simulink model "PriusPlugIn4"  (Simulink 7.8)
settings: Solver=ode23t  StartTime=0.0  StopTime=1180  MaxStep=0.01  RelTol=1e-3
InitFcn:
  | init_Prius_GT
StopFcn:
  | Vyhodnoceni
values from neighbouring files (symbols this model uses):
  k = Nr/Ns    (= 2.6)    [init_Prius_GT.m]
  Mpr = Nr/(Nr+Ns)    (= 0.722222222222)    [init_Prius_GT.m]
  Mps = Ns/(Nr+Ns)    (= 0.277777777778)    [init_Prius_GT.m]
  om_diff_ic = 0    [init_Prius_GT.m]
  omric = 0    [init_Prius_GT.m]
  rpm_FMEP = [1,500,1000,1500,2000,2500,3000,3500,4000,4500,5000]    [init_Prius_GT.m]
  t_sample = 0.1    [init_Prius_GT.m]
  torque_FMEP = [0,0,0.58,0.66,0.75,0.84,0.93,1.1,1.3,1.4,1.5].*(Vdis/(4*pi))*100000    [init_Prius_GT.m]
  vf0 = 0    [init_Prius_GT.m]
undefined symbols (not defined in the file or in its folder): Battery, Battery_Pack, Clutch, Differential, Driveshaft, Engine, Environment, Gearbox, Motor, Powertrain, table_FMEP, Vehicle
libraries: simulink x24, simulink_extras x4, simulink_need_slupdate x1
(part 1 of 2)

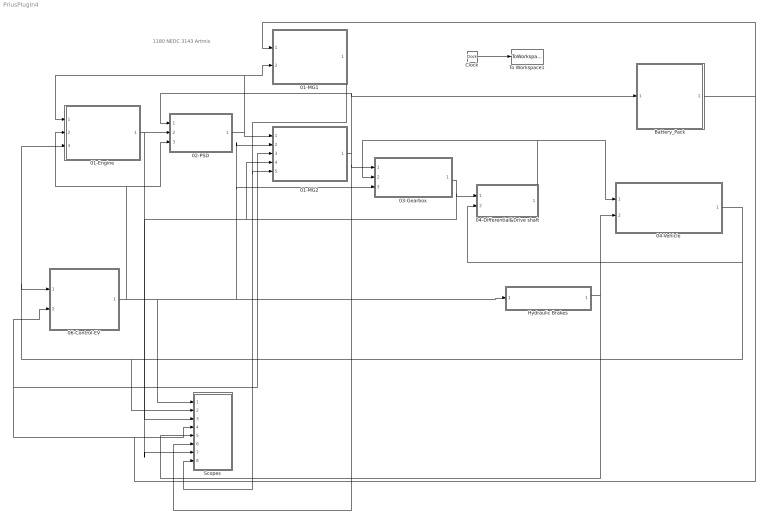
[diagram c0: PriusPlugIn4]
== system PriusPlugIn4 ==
  note: 1180 NEDC 3143 Artmis
  01-Engine : Subsystem  AncestorBlock=Powertrain/01-Engine
  01-MG1 : Subsystem  AncestorBlock=Powertrain/Electric Drive
  01-MG2 : Subsystem  AncestorBlock=Powertrain/Electric Drive
  02-PSD : Subsystem  AncestorBlock=Powertrain/02-Clutch
  03-Gearbox : Subsystem  AncestorBlock=Powertrain/03-Gearbox
  04-Differential&Drive shaft : Subsystem  AncestorBlock=Powertrain/04-Differential&Drive shaft
  04-Vehicle : Subsystem  AncestorBlock=Powertrain/05-Vehicle
  06-Control-EV : Subsystem
  Battery_Pack : Subsystem  AncestorBlock=Powertrain/Battery_Pack
  Clock : Clock
  Hydraulic Brakes : Subsystem  AncestorBlock=Powertrain/Hydraulic Brakes  TreatAsAtomicUnit=on
  Scopes : Subsystem
  To Workspace1 : ToWorkspace  VariableName=t  SampleTime=t_sample  SaveFormat=Array
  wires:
  03-Gearbox/1(BUS_Gearbox) -> 04-Differential&Drive shaft/1(BUS_Gearbox), Scopes/3(BUS_Gearbox), 01-MG2/4(BUS_Gearbox)
  04-Differential&Drive shaft/1(BUS_Driveshaft) -> 03-Gearbox/2(BUS_Driveshaft), 04-Vehicle/1(BUS_Driveshaft_Front)
  06-Control-EV/1(BUS_Control) -> Scopes/1(BUS_Control), 03-Gearbox/3(BUS_Control), 01-MG2/2(BUS_Control), Hydraulic Brakes/1(BUS_Control), 01-Engine/2(BUS_Control), 02-PSD/3(BUS_Control)
  04-Vehicle/1(BUS_Vehicle) -> 04-Differential&Drive shaft/2(BUS_Vehicle), Scopes/2(BUS_Vehicle), 06-Control-EV/1(BUS_Vehicle), 01-Engine/3(BUS_vehicle)
  Battery_Pack/1(BUS_Battery) -> Scopes/4(BUS_Battery), 06-Control-EV/2(BUS_Battery), 01-MG2/3(BUS_Battery), 01-MG1/1(BUS_Battery)
  Hydraulic Brakes/1(BUS_Brakes) -> Scopes/5(BUS_Brakes), 04-Vehicle/2(BUS_Brakes)
  01-Engine/1(BUS_Engine) -> 02-PSD/2(BUS_Engine), Scopes/7(BUS_Engine)
  02-PSD/1(BUS_PSD) -> 01-MG2/1(BUS_PSD), 01-Engine/1(BUS_PSD), 01-MG1/2(BUS_PSD)
  01-MG2/1(BUS_MG2) -> 02-PSD/1(BUS_MG2), Battery_Pack/1(BUS_MG2), 03-Gearbox/1(BUS_MG2), Scopes/6(BUS_Motor)
  01-MG1/1(BUS_MG1) -> 01-MG2/5(BUS_MG1), Scopes/8(BUS_MG1)
  Clock/1 -> To Workspace1/1

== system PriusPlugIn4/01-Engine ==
  BUS_PSD : Inport
  BUS_Control : Inport  Port=2
  BUS_vehicle : Inport  Port=3
  1-D Lookup Table : Lookup_n-D  NumberOfTableDimensions=1  BreakpointsForDimension1=[1000,1625,2250,3000,3750,4500,5250,5625]  Table=[85,90,100,112,100,92,85,78]  RndMeth=Simplest
  Bus Creator : BusCreator  Inputs=6
  Bus Selector : BusSelector  OutputSignals=om_c
  Bus Selector1 : BusSelector  OutputSignals=Throttle_Engine[-],Throttle_excd,Mode
  Bus Selector2 : BusSelector  OutputSignals=s_veh
  Consumption/Emissions : Subsystem
  Display : Display
  Mechanical : Subsystem
  Mux : Mux  Inputs=2
  Product2 : Product
  Saturation : Saturate  UpperLimit=inf  LowerLimit=0
  Scope : Scope  NumInputPorts=3
  Scope1 : Scope
  rad2rpm : Gain  Gain=30/pi
  BUS_Engine : Outport
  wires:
  Product2/1 -> Mux/1, Mechanical/1(Te_dem), Scope/3
  1-D Lookup Table/1 -> Product2/1
  Bus Selector1/1 -> Scope/1, Product2/2  "<Throttle_Engine[-]>"
  Consumption/Emissions/2(Fuel_cons_m) -> Bus Creator/5  "Fuel_cons_m"
  Saturation/1 -> Consumption/Emissions/2(Pe)
  Consumption/Emissions/1(Fuel_cons) -> Bus Creator/4  "fuel_cons [l_100km]"
  Bus Selector2/1 -> Display/1, Consumption/Emissions/3(s)  "<s_veh>"
  BUS_vehicle/1 -> Bus Selector2/1
  BUS_Control/1 -> Bus Selector1/1
  Bus Selector/1 -> Mechanical/2(om_fric)  "<om_c>"
  BUS_PSD/1 -> Bus Selector/1
  Bus Creator/1 -> BUS_Engine/1
  Mechanical/3(Tec) -> Mux/2, Consumption/Emissions/4(Te), Bus Creator/3  "Teng [Nm]"
  Mechanical/2(Pe) -> Saturation/1, Bus Creator/2  "Pe[kW]"
  Mechanical/1(om_e) -> rad2rpm/1
  rad2rpm/1 -> 1-D Lookup Table/1, Scope/2, Bus Creator/1, Consumption/Emissions/1(n_eng[rpm])  "n_eng[rpm]"
  Mechanical/4(Pe_dem) -> Bus Creator/6  "Pe_dem[kW]"
  Bus Selector1/2 -> Mechanical/3(Multip)  "<Throttle_excd>"
  Mux/1 -> Scope1/1

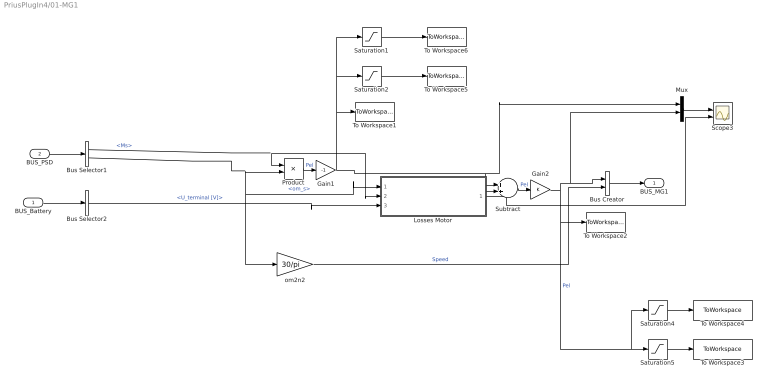
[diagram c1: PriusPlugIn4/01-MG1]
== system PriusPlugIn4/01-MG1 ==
  BUS_Battery : Inport
  BUS_PSD : Inport  Port=2
  Bus Creator : BusCreator  Inputs=2
  Bus Selector1 : BusSelector  OutputSignals=Ms,om_s
  Bus Selector2 : BusSelector  OutputSignals=U_terminal [V]
  Gain1 : Gain  Gain=-1
  Gain2 : Gain
  Losses Motor : Subsystem
  Mux : Mux  Inputs=2
  Product : Product
  Saturation1 : Saturate  UpperLimit=0  LowerLimit=-inf
  Saturation2 : Saturate  UpperLimit=inf  LowerLimit=0
  Saturation4 : Saturate  UpperLimit=0  LowerLimit=-inf
  Saturation5 : Saturate  UpperLimit=inf  LowerLimit=0
  Scope3 : Scope  NumInputPorts=2
  Subtract : Sum
  To Workspace1 : ToWorkspace  VariableName=P_MG1  SampleTime=t_sample  SaveFormat=Array
  To Workspace2 : ToWorkspace  VariableName=P_MG1el  SampleTime=t_sample  SaveFormat=Array
  To Workspace3 : ToWorkspace  VariableName=P_MG1el_mot  SampleTime=t_sample  SaveFormat=Array
  To Workspace4 : ToWorkspace  VariableName=P_MG1el_gen  SampleTime=t_sample  SaveFormat=Array
  To Workspace5 : ToWorkspace  VariableName=P_MG1mech_mot  SampleTime=t_sample  SaveFormat=Array
  To Workspace6 : ToWorkspace  VariableName=P_MG1mech_gen  SampleTime=t_sample  SaveFormat=Array
  om2n2 : Gain  Gain=30/pi
  BUS_MG1 : Outport
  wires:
  BUS_Battery/1 -> Bus Selector2/1
  BUS_PSD/1 -> Bus Selector1/1
  Bus Selector1/1 -> Losses Motor/2(Torque), Product/1  "<Ms>"
  Bus Selector1/2 -> Losses Motor/1(Speed), om2n2/1, Product/2  "<om_s>"
  Product/1 -> Gain1/1  "Pel"
  Bus Creator/1 -> BUS_MG1/1
  Subtract/1 -> Gain2/1  "Pel"
  Losses Motor/1(P_loss) -> Scope3/2, Subtract/2
  Gain1/1 -> Saturation1/1, Saturation2/1, To Workspace1/1, Mux/1, Subtract/1
  om2n2/1 -> Bus Creator/2  "Speed"
  Saturation4/1 -> To Workspace4/1
  Saturation5/1 -> To Workspace3/1
  Saturation1/1 -> To Workspace6/1
  Saturation2/1 -> To Workspace5/1
  Mux/1 -> Scope3/1
  Bus Selector2/1 -> Losses Motor/3(Voltage [V])  "<U_terminal [V]>"
  Gain2/1 -> Mux/2, Bus Creator/1, Saturation4/1, Saturation5/1, To Workspace2/1  "Pel"

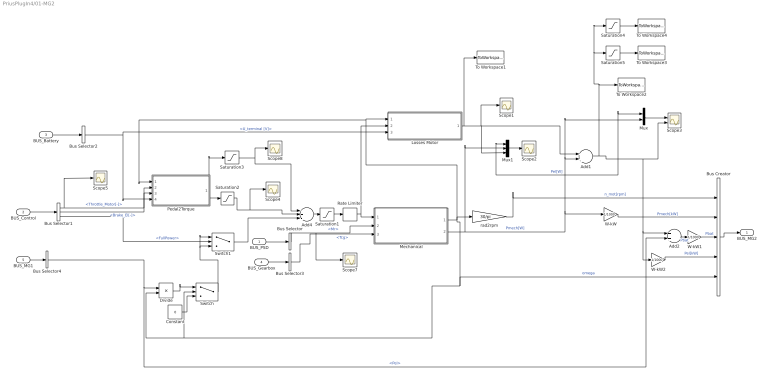
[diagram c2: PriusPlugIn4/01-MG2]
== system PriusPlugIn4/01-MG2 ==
  BUS_PSD : Inport
  BUS_Control : Inport  Port=2
  BUS_Battery : Inport  Port=3
  BUS_Gearbox : Inport  Port=4
  BUS_MG1 : Inport  Port=5
  Add1 : Sum
  Add2 : Sum
  Add4 : Sum  Inputs=++-
  Bus Creator : BusCreator  Inputs=5
  Bus Selector : BusSelector  OutputSignals=Mr
  Bus Selector1 : BusSelector  OutputSignals=Throttle_Motor[-],Brake_El[-],FullPower
  Bus Selector2 : BusSelector  OutputSignals=U_terminal [V]
  Bus Selector3 : BusSelector  OutputSignals=Tcg
  Bus Selector4 : BusSelector  OutputSignals=Pel
  Constant : Constant  Value=0
  Divide : Product  Inputs=*/
  Losses Motor : Subsystem
  Mechanical : Subsystem
  Mux : Mux  Inputs=2
  Mux1 : Mux  Inputs=3
  Pedal2Torque : Subsystem
  Rate Limiter : RateLimiter  RisingSlewLimit=100  FallingSlewLimit=-100  SampleTimeMode=inherited
  Saturation1 : Saturate  UpperLimit=500  LowerLimit=-500
  Saturation2 : Saturate  UpperLimit=inf  LowerLimit=0
  Saturation3 : Saturate  UpperLimit=0  LowerLimit=-inf
  Saturation4 : Saturate  UpperLimit=0  LowerLimit=-inf
  Saturation5 : Saturate  UpperLimit=inf  LowerLimit=0
  Scope{1..2,4..5,7..8} (6 alike) : Scope
  Scope3 : Scope  NumInputPorts=2
  Switch : Switch  Threshold=3
  Switch1 : Switch  Threshold=1
  To Workspace1 : ToWorkspace  VariableName=P_MG2_loss  SampleTime=t_sample  SaveFormat=Array
  To Workspace2 : ToWorkspace  VariableName=P_MG2el  SampleTime=t_sample  SaveFormat=Array
  To Workspace3 : ToWorkspace  VariableName=P_MG2el_mot  SampleTime=t_sample  SaveFormat=Array
  To Workspace4 : ToWorkspace  VariableName=P_MG2el_gen  SampleTime=t_sample  SaveFormat=Array
  W-kW : Gain  Gain=1/1000
  W-kW1 : Gain  Gain=1/1000
  W-kW2 : Gain  Gain=1/1000
  rad2rpm : Gain  Gain=30/pi
  BUS_MG2 : Outport
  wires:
  W-kW2/1 -> Bus Creator/4  "Pel[kW]"
  W-kW/1 -> Bus Creator/2  "Pmech[kW]"
  Bus Selector1/2 -> Pedal2Torque/3(Brake_el[-])  "<Brake_El[-]>"
  Bus Selector1/1 -> Pedal2Torque/2(Throttle_pedal[-]), Scope5/1  "<Throttle_Motor[-]>"
  BUS_Control/1 -> Bus Selector1/1
  BUS_PSD/1 -> Bus Selector/1
  Bus Creator/1 -> BUS_MG2/1
  Mechanical/2(Pmech) -> W-kW/1, Mux/2, Add1/2, Mux1/2  "Pmech[W]"
  Mechanical/1(om_e) -> Divide/2, Switch/2, Bus Creator/5, rad2rpm/1, Losses Motor/1(Speed), Pedal2Torque/1(om_motor)  "omega"
  rad2rpm/1 -> Bus Creator/1  "n_mot[rpm]"
  BUS_Battery/1 -> Bus Selector2/1
  Bus Selector2/1 -> Losses Motor/3(Voltage [V]), Pedal2Torque/4(Voltage [V])  "<U_terminal [V]>"
  Losses Motor/1(P_loss) -> To Workspace1/1, Mux1/3, Add1/1, Scope1/1
  BUS_Gearbox/1 -> Bus Selector3/1
  Bus Selector3/1 -> Mechanical/3(Tcg)  "<Tcg>"
  Bus Selector/1 -> Mechanical/2(Tr), Scope7/1  "<Mr>"
  BUS_MG1/1 -> Bus Selector4/1
  Add1/1 -> To Workspace2/1, Saturation4/1, Saturation5/1, Mux1/1, Mux/1, Scope3/2, Add2/1, W-kW2/1  "Pel[W]"
  Mux/1 -> Scope3/1
  Pedal2Torque/1(Te) -> Saturation2/1, Saturation3/1
  Saturation3/1 -> Add4/1, Scope8/1
  Add4/1 -> Saturation1/1
  Saturation2/1 -> Add4/2, Scope4/1
  Saturation1/1 -> Rate Limiter/1
  Bus Selector4/1 -> Add2/2, Divide/1  "<Pel>"
  Constant/1 -> Switch/3
  Divide/1 -> Switch/1
  Bus Selector1/3 -> Switch1/2  "<FullPower>"
  Switch/1 -> Switch1/3, Switch1/1
  Switch1/1 -> Add4/3
  Rate Limiter/1 -> Mechanical/1(T_MG2), Losses Motor/2(Torque)
  Add2/1 -> W-kW1/1  "Pbat"
  W-kW1/1 -> Bus Creator/3  "Pbat"
  Mux1/1 -> Scope2/1
  Saturation4/1 -> To Workspace4/1
  Saturation5/1 -> To Workspace3/1

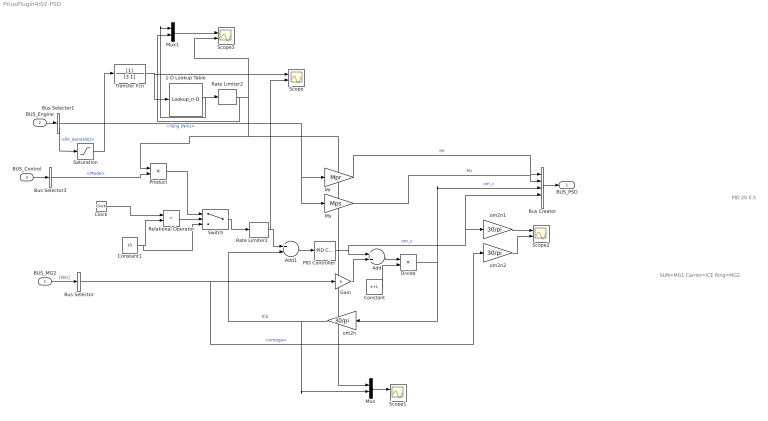
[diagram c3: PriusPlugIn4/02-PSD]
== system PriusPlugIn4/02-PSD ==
  note: SUN=MG1 Carrier=ICE Ring=MG2
  note: PID 20 0.5
  BUS_MG2 : Inport
  BUS_Engine : Inport  Port=2
  BUS_Control : Inport  Port=3
  1-D Lookup Table : Lookup_n-D  NumberOfTableDimensions=1  BreakpointsForDimension1=|  Table=|  RndMeth=Simplest
      | [0
      | 1000
      | 7891
      | 19181
      | 30174
      | 42286
      | 54998]/1000
      | [0
      | 1150
      | 1155
      | 2000
      | 2750
      | 3500
      | 4250]
  Add : Sum
  Add1 : Sum  Inputs=+-
  Bus Creator : BusCreator  Inputs=5
  Bus Selector : BusSelector  OutputSignals=omega
  Bus Selector1 : BusSelector  OutputSignals=n_eng[rpm],Teng [Nm],Pe_dem[kW]
  Bus Selector3 : BusSelector  OutputSignals=Mode
  Clock : Clock
  Constant : Constant  Value=k+1
  Constant1 : Constant  Value=10
  Divide : Product  Inputs=*/
  Gain : Gain  Gain=k
  Mr : Gain  Gain=Mpr
  Ms : Gain  Gain=Mps
  Mux : Mux  Inputs=2
  Mux1 : Mux  Inputs=2
  PID Controller : simulink/Continuous/PID Controller  Controller=PID  TimeDomain=Continuous-time  SampleTime=1  IntegratorMethod=Forward Euler  FilterMethod=Forward Euler  Form=Parallel  P=20  I=0.5*10  D=0  N=0  InitialConditionSource=internal  InitialConditionForIntegrator=0  InitialConditionForFilter=0  ExternalReset=none  LimitOutput=off  UpperSaturationLimit=6500/30*pi  LowerSaturationLimit=-6500/30*pi  LinearizeAsGain=off  AntiWindupMode=none  Kb=1  TrackingMode=off  Kt=1  PParamMin=[]  PParamMax=[]  IParamMin=[]  IParamMax=[]  DParamMin=[]  DParamMax=[]  NParamMin=[]  NParamMax=[]  KbParamMin=[]  KbParamMax=[]  KtParamMin=[]  KtParamMax=[]  POutMin=[]  POutMax=[]  IOutMin=[]  IOutMax=[]  DOutMin=[]  DOutMax=[]  NOutMin=[]  NOutMax=[]  KbOutMin=[]  KbOutMax=[]  KtOutMin=[]  KtOutMax=[]  IntegratorOutMin=[]  IntegratorOutMax=[]  FilterOutMin=[]  FilterOutMax=[]  SumOutMin=[]  SumOutMax=[]  SumI1OutMin=[]  SumI1OutMax=[]  SumI2OutMin=[]  SumI2OutMax=[]  SumI3OutMin=[]  SumI3OutMax=[]  SumDOutMin=[]  SumDOutMax=[]  SaturationOutMin=[]  SaturationOutMax=[]  IntegratorContinuousStateAttributes=''  IntegratorStateMustResolveToSignalObject=off  IntegratorRTWStateStorageClass=Auto  FilterContinuousStateAttributes=''  FilterStateMustResolveToSignalObject=off  FilterRTWStateStorageClass=Auto
  Product : Product
  Rate Limiter1 : RateLimiter  RisingSlewLimit=300  FallingSlewLimit=-300
  Rate Limiter2 : RateLimiter  RisingSlewLimit=500  FallingSlewLimit=-500
  Relational Operator : RelationalOperator  Operator=>  OutDataTypeStr=boolean
  Saturation : Saturate  UpperLimit=47  LowerLimit=0
  Scope{,1..3} (4 alike) : Scope  NumInputPorts=2
  Switch : Switch
  Transfer Fcn : TransferFcn  Denominator=[3 1]
  om2n : Gain  Gain=30/pi
  om2n1 : Gain  Gain=30/pi
  om2n2 : Gain  Gain=30/pi
  BUS_PSD : Outport
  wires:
  BUS_Engine/1 -> Bus Selector1/1
  Bus Creator/1 -> BUS_PSD/1
  BUS_MG2/1 -> Bus Selector/1  "[Nm]"
  BUS_Control/1 -> Bus Selector3/1
  Bus Selector1/2 -> Mr/1, Ms/1  "<Teng [Nm]>"
  PID Controller/1 -> Add/1, Bus Creator/4, om2n1/1  "om_s"
  Gain/1 -> Add/2
  Add/1 -> Divide/1
  Constant/1 -> Divide/2
  Divide/1 -> Bus Creator/3, om2n/1  "om_c"
  Mr/1 -> Bus Creator/1  "Mr"
  om2n/1 -> Add1/2, Mux/2  "ICE"
  Add1/1 -> PID Controller/1
  Ms/1 -> Bus Creator/2  "Ms"
  Bus Selector/1 -> Gain/1, om2n2/1  "<omega>"
  Constant1/1 -> Relational Operator/2, Switch/3
  Clock/1 -> Relational Operator/1
  Relational Operator/1 -> Switch/2
  Switch/1 -> Rate Limiter1/1
  Bus Selector1/3 -> Saturation/1  "<Pe_dem[kW]>"
  1-D Lookup Table/1 -> Mux1/1, Rate Limiter2/1
  Mux/1 -> Scope1/1
  Product/1 -> Switch/1
  Rate Limiter1/1 -> Add1/1, Scope/2
  om2n1/1 -> Scope2/1
  om2n2/1 -> Scope2/2
  Bus Selector3/1 -> Product/2  "<Mode>"
  Saturation/1 -> Transfer Fcn/1
  Mux1/1 -> Scope3/1
  Rate Limiter2/1 -> Mux1/2, Product/1, Mux/1, Scope3/2
  Transfer Fcn/1 -> Scope/1, 1-D Lookup Table/1

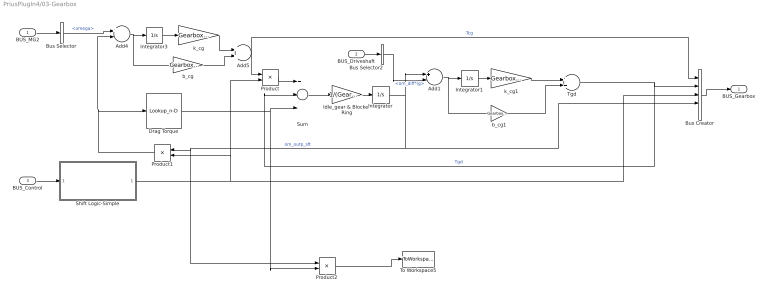
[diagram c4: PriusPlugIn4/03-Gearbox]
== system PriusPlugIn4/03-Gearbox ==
  BUS_MG2 : Inport
  BUS_Driveshaft : Inport  Port=2
  BUS_Control : Inport  Port=3
  Add1 : Sum  Inputs=+-
  Add4 : Sum  Inputs=+-
  Add5 : Sum
  Bus Creator : BusCreator  Inputs=5
  Bus Selector : BusSelector  OutputSignals=omega
  Bus Selector2 : BusSelector  OutputSignals=om_diff*ig
  Drag Torque : Lookup_n-D  NumberOfTableDimensions=1  BreakpointsForDimension1=[0 100 200 300 400]  Table=[0 1 2 3 3.5]  RndMeth=Simplest
  Idle_gear & Blocker Ring : Gain  Gain=1/(Gearbox.Inpsft.Inertia+Gearbox.Outpsft.Inertia)
  Integrator : Integrator
  Integrator1 : Integrator
  Integrator3 : Integrator
  Product : Product
  Product1 : Product
  Product2 : Product
  Shift Logic-Simple : Subsystem
  Sum : Sum  Inputs=+--
  Tgd : Sum
  To Workspace5 : ToWorkspace  VariableName=P_Gearbox  SampleTime=t_sample  SaveFormat=Array
  b_cg : Gain  Gain=Gearbox.Inpsft.b
  b_cg1 : Gain  Gain=Gearbox.Outpsft.b
  k_cg : Gain  Gain=Gearbox.Inpsft.c
  k_cg1 : Gain  Gain=Gearbox.Outpsft.c
  BUS_Gearbox : Outport
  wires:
  Bus Selector2/1 -> Add1/2  "<om_diff*ig>"
  BUS_Driveshaft/1 -> Bus Selector2/1
  Tgd/1 -> Bus Creator/2, Sum/2  "Tgd"
  Add1/1 -> b_cg1/1, Integrator1/1
  Integrator1/1 -> k_cg1/1
  k_cg1/1 -> Tgd/1
  b_cg1/1 -> Tgd/2
  Shift Logic-Simple/1(Gear_ratio) -> Bus Creator/3, Product1/2, Product/2
  Bus Creator/1 -> BUS_Gearbox/1
  BUS_Control/1 -> Shift Logic-Simple/1(BUS_Control)
  Bus Selector/1 -> Add4/1  "<omega>"
  BUS_MG2/1 -> Bus Selector/1
  Product1/1 -> Drag Torque/1, Add4/2
  Product/1 -> Sum/1
  b_cg/1 -> Add5/2
  k_cg/1 -> Add5/1
  Integrator3/1 -> k_cg/1
  Add4/1 -> Integrator3/1, b_cg/1
  Integrator/1 -> Add1/1, Product2/1, Product1/1, Bus Creator/4  "om_outp_sft"
  Idle_gear & Blocker Ring/1 -> Integrator/1
  Sum/1 -> Idle_gear & Blocker Ring/1
  Add5/1 -> Bus Creator/1, Product/1  "Tcg"
  Product2/1 -> To Workspace5/1
  Drag Torque/1 -> Product2/2, Sum/3

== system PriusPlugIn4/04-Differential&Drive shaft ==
  BUS_Gearbox : Inport
  BUS_Vehicle : Inport  Port=2
  Bus Creator : BusCreator  Inputs=2
  Bus Selector2 : BusSelector  OutputSignals=Tgd
  Differential : Subsystem
  Driveshafts : Subsystem
  BUS_Driveshaft : Outport
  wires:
  Driveshafts/1(T_drvsft) -> Differential/2(T_drv_sft), Bus Creator/1
  Differential/2(om_diff*ig) -> Bus Creator/2  "om_diff*ig"
  Bus Selector2/1 -> Differential/1(Tgd)  "<Tgd>"
  Differential/1(om_diff) -> Driveshafts/1(om_diff)
  BUS_Vehicle/1 -> Driveshafts/2(BUS_Vehicle)
  Bus Creator/1 -> BUS_Driveshaft/1
  BUS_Gearbox/1 -> Bus Selector2/1

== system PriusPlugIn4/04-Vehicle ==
  BUS_Driveshaft_Front : Inport
  BUS_Brakes : Inport  Port=2
  "          1" : Product  Inputs=**
  "          2" : Product  Inputs=**
  Add : Sum
  Bus Creator : BusCreator  Inputs=5
  Bus Selector1 : BusSelector  OutputSignals=T_drvsft
  Bus Selector3 : BusSelector  OutputSignals=Brakes_Front,Brakes_Rear
  Dynamics : Subsystem
  Subtract2 : Sum
  Tire front : Subsystem
  Tire rear : Subsystem
  To Workspace2 : ToWorkspace  VariableName=P_brakes  SampleTime=t_sample  SaveFormat=Array
  Weight distribution : Subsystem
  BUS_Vehicle : Outport
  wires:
  "          2"/1 -> Subtract2/2
  Subtract2/1 -> To Workspace2/1
  "          1"/1 -> Subtract2/1
  Bus Selector3/2 -> Tire rear/2(T_drsft), "          2"/2  "<Brakes_Rear>"
  Bus Selector3/1 -> "          1"/2, Add/2  "<Brakes_Front>"
  BUS_Brakes/1 -> Bus Selector3/1
  Bus Selector1/1 -> Add/1  "<T_drvsft>"
  Add/1 -> Tire front/2(T_drsft)
  Dynamics/2(s_veh) -> Bus Creator/2  "s_veh"
  Tire front/1(F_tire) -> Dynamics/1(F_tire_front)
  Tire rear/1(F_tire) -> Dynamics/2(F_tire_rear)
  BUS_Driveshaft_Front/1 -> Bus Selector1/1
  Bus Creator/1 -> BUS_Vehicle/1
  Weight distribution/1(Fn_Wheel_F) -> Dynamics/3(Fn_Wheel_F)
  Weight distribution/2(Fn_Wheel_R) -> Dynamics/4(Fn_Wheel_R)
  Dynamics/1(v_veh) -> Bus Creator/1  "v_veh"
  Dynamics/3(v_f[m/s]) -> Tire front/1(v_f), Tire rear/1(v_f)
  Dynamics/4(Acc) -> Bus Creator/5, Weight distribution/1(acc)  "a_veh"
  Tire front/2(om_wheel) -> "          1"/1, Bus Creator/3  "om_wheel_f"
  Tire rear/2(om_wheel) -> "          2"/1, Bus Creator/4  "om_wheel_r"

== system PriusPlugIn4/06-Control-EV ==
  BUS_Vehicle : Inport
  BUS_Battery : Inport  Port=2
  Brakes : Scope  NumInputPorts=5
  Bus Creator : BusCreator  Inputs=10
  Bus Selector1 : BusSelector  OutputSignals=SOC[%]
  Bus Selector2 : BusSelector  OutputSignals=v_veh,a_veh
  Cockpit : Subsystem
  Constant : Constant  Value=0
  Cycle : Subsystem
  Driver : Subsystem
  Electric : Subsystem
  Full Power : Subsystem
  Gain : Gain  Gain=0
  Hybrid : Subsystem
  Manual Switch : simulink/Signal Routing/Manual Switch  sw=0  action=0  varsize=off
  BUS_Control : Outport
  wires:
  Cockpit/2(Clutch1) -> Bus Creator/2  "Clutch_pedal[-]"
  Cockpit/1(ThrottleEngine) -> Bus Creator/1  "Throttle_Engine[-]"
  Cockpit/3(BrakeEl) -> Bus Creator/3  "Brake_El[-]"
  Driver/1(Throttle [Nm]) -> Cockpit/1(Throttle_in), Electric/3(Throttle), Hybrid/3(Throttle), Full Power/3(Throttle)
  Driver/2(Brake [Nm]) -> Cockpit/2(Brake)
  Cycle/2(v_dem [-]) -> Bus Creator/5, Driver/2(v_dem [km/h])  "v_dem[kmh]"
  Cycle/1(Gear_dem [-]) -> Bus Creator/4  "Gear[-]"
  Bus Creator/1 -> BUS_Control/1
  BUS_Vehicle/1 -> Bus Selector2/1
  Bus Selector2/1 -> Cockpit/4(v-veh), Driver/1(v_veh [km/h]), Hybrid/1(In1), Full Power/1(In1), Electric/1(v_veh)  "<v_veh>"
  Bus Selector2/2 -> Cockpit/3(a-veh)  "<a_veh>"
  Cockpit/4(BrakeHyd) -> Bus Creator/6  "Brake_Hyd[-]"
  Cockpit/5(ThrottleMotor) -> Bus Creator/7  "Throttle_Motor[-]"
  BUS_Battery/1 -> Bus Selector1/1
  Bus Selector1/1 -> Electric/2(SOC), Hybrid/2(SOC), Full Power/2(SOC)  "<SOC[%]>"
  Electric/1(Out1) -> Brakes/1  "Electric"
  Hybrid/1(Out1) -> Brakes/2, Manual Switch/2  "Mode"
  Full Power/1(Out1) -> Gain/1  "FullPower"
  Driver/3(Throttle_excd) -> Bus Creator/10  "Throttle_excd"
  Manual Switch/1 -> Cockpit/5(Mode), Bus Creator/8  "Mode"
  Constant/1 -> Manual Switch/1
  Gain/1 -> Cockpit/6(FullPower), Brakes/3, Bus Creator/9  "FullPower"

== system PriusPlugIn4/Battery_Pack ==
  BUS_MG2 : Inport
  Bus Creator : BusCreator  Inputs=5
  Bus Selector : BusSelector  OutputSignals=Pbat
  Cell : Subsystem
  Divide : Product  Inputs=*/
  Divide1 : Product  Inputs=*/
  Gain1 : Gain  Gain=1000
  Memory1 : Memory  X0=400
  Memory2 : Memory
  N_Cells_P : Constant
  N_Cells_S : Constant  Value=100
  Product1 : Product
  Product2 : Product  Inputs=3
  To Workspace1 : ToWorkspace  VariableName=SOC  SampleTime=t_sample  SaveFormat=Array
  To Workspace2 : ToWorkspace  VariableName=P_Batt_loss  SampleTime=t_sample  SaveFormat=Array
  BUS_Battery : Outport
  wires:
  Memory1/1 -> Divide/2
  Cell/4(T_cell[C]) -> Bus Creator/5  "T_cell[C]"
  Product2/1 -> Bus Creator/4, To Workspace2/1  "P_loss [W]"
  Cell/3(SOC[%]) -> Bus Creator/3, To Workspace1/1  "SOC[%]"
  Divide1/1 -> Cell/1(Current [A])
  N_Cells_P/1 -> Product2/3, Divide1/2
  Divide/1 -> Divide1/1, Bus Creator/2  "Current [A]"
  Cell/2(P_loss [w]) -> Product2/1
  N_Cells_S/1 -> Product2/2, Product1/1
  Cell/1(U_terminal [V]) -> Product1/2
  Product1/1 -> Memory1/1, Bus Creator/1  "U_terminal [V]"
  Gain1/1 -> Divide/1
  BUS_MG2/1 -> Bus Selector/1
  Bus Creator/1 -> BUS_Battery/1
  Memory2/1 -> Gain1/1
  Bus Selector/1 -> Memory2/1  "<Pbat>"

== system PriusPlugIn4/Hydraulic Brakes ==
  BUS_Control : Inport
  Bus Creator : BusCreator  Inputs=2
  Bus Selector : BusSelector  OutputSignals=Brake_Hyd[-]
  Gain1 : Gain  Gain=0.6
  Gain2 : Gain  Gain=0.4
  Pos2Nm : Gain  Gain=800
  BUS_Brakes : Outport
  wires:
  Bus Selector/1 -> Pos2Nm/1  "<Brake_Hyd[-]>"
  BUS_Control/1 -> Bus Selector/1
  Gain1/1 -> Bus Creator/1  "Brakes_Front"
  Gain2/1 -> Bus Creator/2  "Brakes_Rear"
  Bus Creator/1 -> BUS_Brakes/1
  Pos2Nm/1 -> Gain1/1, Gain2/1

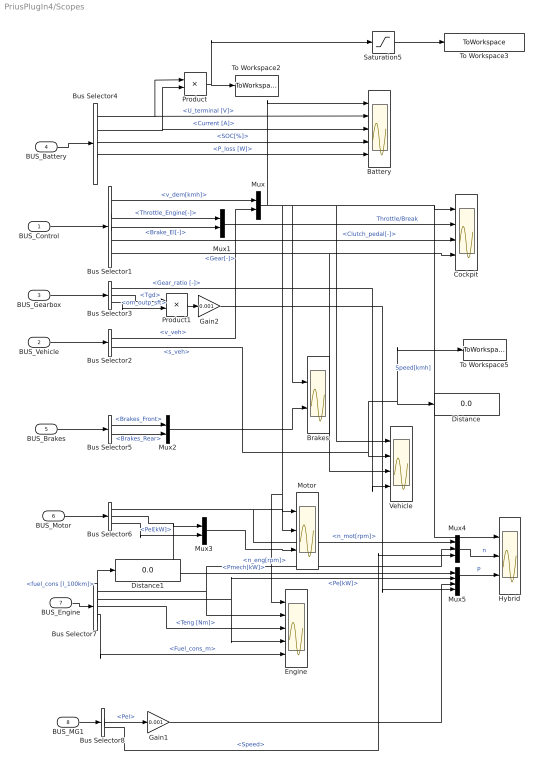
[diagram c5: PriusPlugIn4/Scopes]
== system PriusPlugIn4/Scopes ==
  BUS_Control : Inport
  BUS_Vehicle : Inport  Port=2
  BUS_Gearbox : Inport  Port=3
  BUS_Battery : Inport  Port=4
  BUS_Brakes : Inport  Port=5
  BUS_Motor : Inport  Port=6
  BUS_Engine : Inport  Port=7
  BUS_MG1 : Inport  Port=8
  Battery : Scope  NumInputPorts=5
  Brakes : Scope  NumInputPorts=2
  Bus Selector1 : BusSelector  OutputSignals=v_dem[kmh],Throttle_Engine[-],Brake_El[-],Clutch_pedal[-],Gear[-]
  Bus Selector2 : BusSelector  OutputSignals=v_veh,s_veh
  Bus Selector3 : BusSelector  OutputSignals=Gear_ratio [-],Tgd,om_outp_sft
  Bus Selector4 : BusSelector  OutputSignals=U_terminal [V],Current [A],SOC[%],P_loss [W],T_cell[C]
  Bus Selector5 : BusSelector  OutputSignals=Brakes_Front,Brakes_Rear
  Bus Selector6 : BusSelector  OutputSignals=n_mot[rpm],Pmech[kW],Pel[kW]
  Bus Selector7 : BusSelector  OutputSignals=n_eng[rpm],Pe[kW],Teng [Nm],Fuel_cons_m,fuel_cons [l_100km]
  Bus Selector8 : BusSelector  OutputSignals=Pel,Speed
  Cockpit : Scope  NumInputPorts=4
  Distance : Display
  Distance1 : Display
  Engine : Scope  NumInputPorts=5
  Gain1 : Gain  Gain=0.001
  Gain2 : Gain  Gain=0.001
  Hybrid : Scope  NumInputPorts=3
  Motor : Scope  NumInputPorts=3
  Mux{,1..3} (4 alike) : Mux  Inputs=2
  Mux4 : Mux  Inputs=3
  Mux5 : Mux
  Product : Product
  Product1 : Product
  Saturation5 : Saturate  UpperLimit=inf  LowerLimit=0
  To Workspace2 : ToWorkspace  VariableName=Pbat  SampleTime=t_sample  SaveFormat=Array
  To Workspace3 : ToWorkspace  VariableName=Pbat_pos  SampleTime=t_sample  SaveFormat=Array
  To Workspace5 : ToWorkspace  VariableName=s  SampleTime=t_sample  SaveFormat=Array
  Vehicle : Scope  NumInputPorts=4
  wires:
  BUS_Control/1 -> Bus Selector1/1
  BUS_Vehicle/1 -> Bus Selector2/1
  Bus Selector1/1 -> Mux/1  "<v_dem[kmh]>"
  Bus Selector2/1 -> Mux/2  "<v_veh>"
  Mux/1 -> Vehicle/1, Cockpit/1, Hybrid/1, Brakes/1, Motor/1, Engine/1, Battery/1  "Speed[kmh]"
  Bus Selector1/2 -> Mux1/1  "<Throttle_Engine[-]>"
  Bus Selector1/3 -> Mux1/2  "<Brake_El[-]>"
  Mux1/1 -> Cockpit/2  "Throttle/Break"
  Bus Selector2/2 -> Vehicle/2, Distance/1, To Workspace5/1  "<s_veh>"
  BUS_Gearbox/1 -> Bus Selector3/1
  Bus Selector1/5 -> Vehicle/3, Cockpit/4  "<Gear[-]>"
  Bus Selector1/4 -> Cockpit/3  "<Clutch_pedal[-]>"
  Bus Selector3/1 -> Vehicle/4  "<Gear_ratio [-]>"
  BUS_Battery/1 -> Bus Selector4/1
  Bus Selector4/1 -> Battery/2, Product/1  "<U_terminal [V]>"
  Bus Selector4/2 -> Battery/3, Product/2  "<Current [A]>"
  Bus Selector4/3 -> Battery/4  "<SOC[%]>"
  Bus Selector4/4 -> Battery/5  "<P_loss [W]>"
  BUS_Brakes/1 -> Bus Selector5/1
  Bus Selector5/1 -> Mux2/1  "<Brakes_Front>"
  Bus Selector5/2 -> Mux2/2  "<Brakes_Rear>"
  Mux2/1 -> Brakes/2
  BUS_Motor/1 -> Bus Selector6/1
  Bus Selector6/1 -> Motor/2, Mux4/1  "<n_mot[rpm]>"
  Bus Selector6/2 -> Mux3/1, Mux5/1  "<Pmech[kW]>"
  Bus Selector6/3 -> Mux3/2  "<Pel[kW]>"
  Mux3/1 -> Motor/3
  BUS_Engine/1 -> Bus Selector7/1
  Bus Selector7/1 -> Engine/2, Mux4/2  "<n_eng[rpm]>"
  Bus Selector7/3 -> Engine/3  "<Teng [Nm]>"
  Bus Selector7/2 -> Engine/4, Mux5/2  "<Pe[kW]>"
  Mux4/1 -> Hybrid/2  "n"
  Mux5/1 -> Hybrid/3  "P"
  Product/1 -> Saturation5/1, To Workspace2/1
  Bus Selector7/4 -> Engine/5  "<Fuel_cons_m>"
  BUS_MG1/1 -> Bus Selector8/1
  Bus Selector8/1 -> Gain1/1  "<Pel>"
  Gain1/1 -> Mux5/3
  Bus Selector8/2 -> Mux4/3  "<Speed>"
  Bus Selector7/5 -> Distance1/1  "<fuel_cons [l_100km]>"
  Bus Selector3/2 -> Product1/1  "<Tgd>"
  Bus Selector3/3 -> Product1/2  "<om_outp_sft>"
  Product1/1 -> Gain2/1
  Gain2/1 -> Mux5/4
  Saturation5/1 -> To Workspace3/1

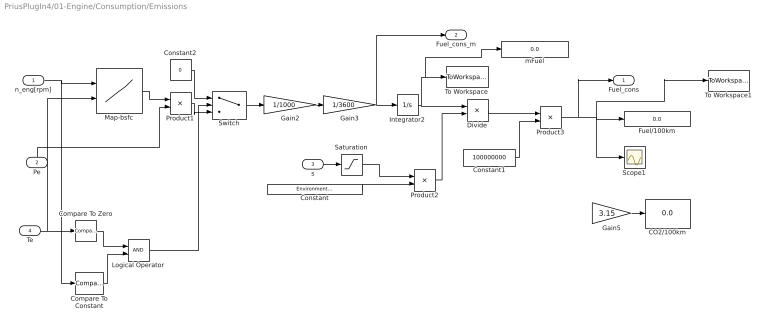
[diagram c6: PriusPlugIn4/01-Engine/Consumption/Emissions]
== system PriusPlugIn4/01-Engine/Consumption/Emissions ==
  n_eng[rpm] : Inport
  Pe : Inport  Port=2
  s : Inport  Port=3
  Te : Inport  Port=4
  CO2/100km : Display
  Compare To Constant : simulink/Logic and Bit Operations/Compare To Constant  relop=>=  const=2000  OutDataTypeStr=uint8
  Compare To Zero : simulink/Logic and Bit Operations/Compare To Zero  relop=<=  OutDataTypeStr=uint8
  Constant : Constant  Value=Environment.Fuel.ro
  Constant1 : Constant  Value=100000000
  Constant2 : Constant  Value=0
  Divide : Product  Inputs=*/
  Fuel/100km : Display
  Gain2 : Gain  Gain=1/1000
  Gain3 : Gain  Gain=1/3600
  Gain5 : Gain  Gain=3.15
  Integrator2 : Integrator
  Logical Operator : Logic  AllPortsSameDT=off  OutDataTypeStr=boolean
  Map-bsfc : Lookup2D  RowIndex=RPM  ColumnIndex=performance  Table=bsfc'  LookUpMeth=Interpolation-Use End Values
  Product1 : Product
  Product2 : Product
  Product3 : Product
  Saturation : Saturate  UpperLimit=inf  LowerLimit=10
  Scope1 : Scope
  Switch : Switch  Threshold=1
  To Workspace : ToWorkspace  VariableName=m_fuel  SampleTime=t_sample  SaveFormat=Array
  To Workspace1 : ToWorkspace  VariableName=fuel_cons_avg  SampleTime=t_sample  SaveFormat=Array
  mFuel : Display
  Fuel_cons : Outport
  Fuel_cons_m : Outport  Port=2
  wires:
  Constant2/1 -> Switch/1
  Switch/1 -> Gain2/1
  Product1/1 -> Switch/3
  Logical Operator/1 -> Switch/2
  Compare To Constant/1 -> Logical Operator/2
  Compare To Zero/1 -> Logical Operator/1
  Te/1 -> Compare To Zero/1, Map-bsfc/2
  Saturation/1 -> Product2/1
  Pe/1 -> Product1/2
  n_eng[rpm]/1 -> Compare To Constant/1, Map-bsfc/1
  Gain5/1 -> CO2/100km/1
  Product3/1 -> To Workspace1/1, Scope1/1, Fuel/100km/1, Fuel_cons/1
  Constant1/1 -> Product3/2
  Divide/1 -> Product3/1
  Product2/1 -> Divide/2
  Constant/1 -> Product2/2
  s/1 -> Saturation/1
  Integrator2/1 -> Divide/1, mFuel/1, To Workspace/1
  Gain3/1 -> Fuel_cons_m/1, Integrator2/1
  Gain2/1 -> Gain3/1
  Map-bsfc/1 -> Product1/1

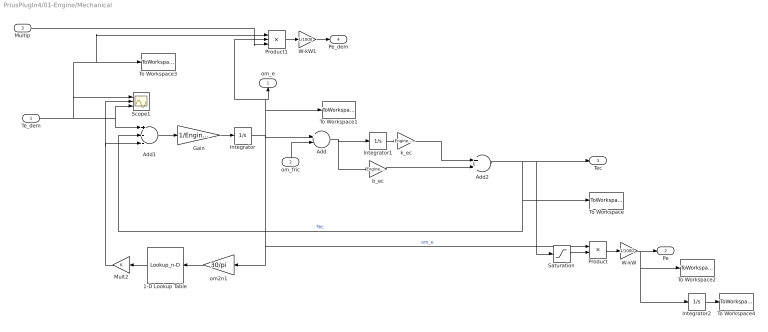
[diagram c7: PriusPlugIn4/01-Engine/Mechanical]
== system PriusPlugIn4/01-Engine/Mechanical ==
  Te_dem : Inport
  om_fric : Inport  Port=2
  Multip : Inport  Port=3
  1-D Lookup Table : Lookup_n-D  NumberOfTableDimensions=1  BreakpointsForDimension1=rpm_FMEP  BreakpointsForDimension2=table_FMEP  Table=torque_FMEP  RndMeth=Simplest
  Add : Sum  Inputs=+-
  Add1 : Sum  Inputs=+--
  Add2 : Sum
  Gain : Gain  Gain=1/Engine.Inertia
  Integrator : Integrator
  Integrator1 : Integrator
  Integrator2 : Integrator
  Mult2 : Gain
  Product : Product
  Product1 : Product  Inputs=3
  Saturation : Saturate  UpperLimit=inf  LowerLimit=0
  Scope1 : Scope  NumInputPorts=3
  To Workspace : ToWorkspace  VariableName=Tengine_f  SampleTime=t_sample  SaveFormat=Array
  To Workspace1 : ToWorkspace  VariableName=om_e_f  SampleTime=t_sample  SaveFormat=Array
  To Workspace2 : ToWorkspace  VariableName=Pe  SampleTime=t_sample  SaveFormat=Array
  To Workspace3 : ToWorkspace  VariableName=Te_dem  SampleTime=t_sample  SaveFormat=Array
  To Workspace4 : ToWorkspace  VariableName=Eengine  SampleTime=t_sample  SaveFormat=Array
  W-kW : Gain  Gain=1/1000
  W-kW1 : Gain  Gain=1/1000
  b_ec : Gain  Gain=Engine.Crankshaft.b
  k_ec : Gain  Gain=Engine.Crankshaft.c
  om2n1 : Gain  Gain=30/pi
  om_e : Outport
  Pe : Outport  Port=2
  Tec : Outport  Port=3
  Pe_dem : Outport  Port=4
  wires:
  W-kW/1 -> Pe/1, Integrator2/1, To Workspace2/1
  Te_dem/1 -> Add1/1, Scope1/3, To Workspace3/1, Product1/1, Scope1/1
  b_ec/1 -> Add2/2
  k_ec/1 -> Add2/1
  Product/1 -> W-kW/1
  om_fric/1 -> Add/2
  Add2/1 -> Saturation/1, Tec/1, To Workspace/1, Add1/2  "Tec"
  Integrator1/1 -> k_ec/1
  Add/1 -> b_ec/1, Integrator1/1
  Integrator/1 -> To Workspace1/1, om_e/1, Product1/2, om2n1/1, Product/1, Add/1  "om_e"
  Gain/1 -> Integrator/1
  Add1/1 -> Gain/1
  Product1/1 -> W-kW1/1
  W-kW1/1 -> Pe_dem/1
  Multip/1 -> Product1/3
  Integrator2/1 -> To Workspace4/1
  1-D Lookup Table/1 -> Mult2/1
  om2n1/1 -> 1-D Lookup Table/1
  Mult2/1 -> Add1/3, Scope1/2
  Saturation/1 -> Product/2

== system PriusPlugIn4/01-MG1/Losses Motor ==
  Speed : Inport
  Torque : Inport  Port=2
  Voltage [V] : Inport  Port=3
  2-D Lookup Table : Lookup_n-D  NumberOfTableDimensions=3  BreakpointsForDimension1=Motor.Maps.vector_speed  BreakpointsForDimension2=Motor.Maps.vector_torque  BreakpointsForDimension3=Motor.Maps.vector_voltage  Table=Motor.Maps.map_ploss  ExtrapMethod=Clip  RemoveProtectionInput=on  UseLastTableValue=on  RndMeth=Simplest
  P_loss : Outport
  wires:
  Speed/1 -> 2-D Lookup Table/1
  Torque/1 -> 2-D Lookup Table/2
  Voltage [V]/1 -> 2-D Lookup Table/3
  2-D Lookup Table/1 -> P_loss/1

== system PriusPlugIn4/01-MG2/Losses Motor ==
  Speed : Inport
  Torque : Inport  Port=2
  Voltage [V] : Inport  Port=3
  2-D Lookup Table : Lookup_n-D  NumberOfTableDimensions=3  BreakpointsForDimension1=Motor.Maps.vector_speed  BreakpointsForDimension2=Motor.Maps.vector_torque  BreakpointsForDimension3=Motor.Maps.vector_voltage  Table=Motor.Maps.map_ploss  ExtrapMethod=Clip  RemoveProtectionInput=on  UseLastTableValue=on  RndMeth=Simplest
  P_loss : Outport
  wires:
  Speed/1 -> 2-D Lookup Table/1
  Torque/1 -> 2-D Lookup Table/2
  Voltage [V]/1 -> 2-D Lookup Table/3
  2-D Lookup Table/1 -> P_loss/1

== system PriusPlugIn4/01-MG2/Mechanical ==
  T_MG2 : Inport
  Tr : Inport  Port=2
  Tcg : Inport  Port=3
  Add1 : Sum  Inputs=++-
  Gain : Gain  Gain=1/Motor.Inertia
  Gain1 : Gain
  Integrator : Integrator
  Mux2 : Mux  Inputs=3
  Product : Product
  Saturation4 : Saturate  UpperLimit=0  LowerLimit=-inf
  Saturation5 : Saturate  UpperLimit=inf  LowerLimit=0
  Scope6 : Scope  NumInputPorts=2
  To Workspace1 : ToWorkspace  VariableName=om_MG2  SampleTime=t_sample  SaveFormat=Array
  To Workspace2 : ToWorkspace  VariableName=P_MG2  SampleTime=t_sample  SaveFormat=Array
  To Workspace3 : ToWorkspace  VariableName=P_MG2mech_mot  SampleTime=t_sample  SaveFormat=Array
  To Workspace4 : ToWorkspace  VariableName=P_MG2mech_gen  SampleTime=t_sample  SaveFormat=Array
  om_e : Outport
  Pmech : Outport  Port=2
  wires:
  T_MG2/1 -> Mux2/1, Product/2, Add1/1
  Integrator/1 -> Product/1, om_e/1, To Workspace1/1  "om_e"
  Gain/1 -> Integrator/1
  Add1/1 -> Mux2/3, Gain/1
  Tcg/1 -> Mux2/2, Add1/3
  Tr/1 -> Gain1/1
  Mux2/1 -> Scope6/1
  Gain1/1 -> Scope6/2, Add1/2
  Product/1 -> Saturation5/1, Saturation4/1, Pmech/1, To Workspace2/1  "Pel[W]"
  Saturation4/1 -> To Workspace4/1
  Saturation5/1 -> To Workspace3/1

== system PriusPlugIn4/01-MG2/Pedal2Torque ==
  om_motor : Inport
  Throttle_pedal[-] : Inport  Port=2
  Brake_el[-] : Inport  Port=3
  Voltage [V] : Inport  Port=4
  1-D Lookup Table : Lookup_n-D  BreakpointsForDimension1=Motor.Maps.vector_speed  BreakpointsForDimension2=Motor.Maps.vector_voltage  Table=Motor.Maps.vector_max_torque  ExtrapMethod=Clip  UseLastTableValue=on  RndMeth=Simplest
  1-D Lookup Table1 : Lookup_n-D  BreakpointsForDimension1=Motor.Maps.vector_speed  BreakpointsForDimension2=Motor.Maps.vector_voltage  Table=Motor.Maps.vector_min_torque  ExtrapMethod=Clip  UseLastTableValue=on  RndMeth=Simplest
  Add : Sum
  Gain : Gain  Gain=-1
  Product1 : Product
  Product2 : Product
  Te : Outport
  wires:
  Gain/1 -> Add/2
  Product1/1 -> Gain/1
  Product2/1 -> Add/1
  1-D Lookup Table1/1 -> Product1/2
  1-D Lookup Table/1 -> Product2/1
  om_motor/1 -> 1-D Lookup Table1/1, 1-D Lookup Table/1
  Add/1 -> Te/1
  Brake_el[-]/1 -> Product1/1
  Voltage [V]/1 -> 1-D Lookup Table1/2, 1-D Lookup Table/2
  Throttle_pedal[-]/1 -> Product2/2

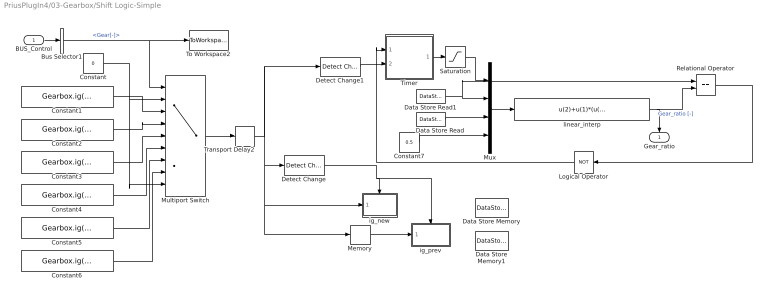
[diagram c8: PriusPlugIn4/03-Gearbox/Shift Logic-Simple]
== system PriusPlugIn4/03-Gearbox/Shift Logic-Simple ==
  BUS_Control : Inport
  Bus Selector1 : BusSelector  OutputSignals=Gear[-]
  Constant : Constant  Value=0
  Constant1 : Constant  Value=Gearbox.ig(1)
  Constant2 : Constant  Value=Gearbox.ig(2)
  Constant3 : Constant  Value=Gearbox.ig(3)
  Constant4 : Constant  Value=Gearbox.ig(4)
  Constant5 : Constant  Value=Gearbox.ig(5)
  Constant6 : Constant  Value=Gearbox.ig(6)
  Constant7 : Constant  Value=0.5
  Data Store Memory : DataStoreMemory  DataStoreName=ig_new
  Data Store Memory1 : DataStoreMemory  DataStoreName=ig_prev
  Data Store Read : DataStoreRead  DataStoreName=ig_new  SampleTime=0
  Data Store Read1 : DataStoreRead  DataStoreName=ig_prev  SampleTime=0
  Detect Change : simulink/Logic and Bit Operations/Detect Change  vinit=0  InputProcessing=Inherited  OutDataTypeStr=uint8
  Detect Change1 : simulink/Logic and Bit Operations/Detect Change  vinit=0  InputProcessing=Inherited  OutDataTypeStr=boolean
  Logical Operator : Logic  Operator=NOT  AllPortsSameDT=off  OutDataTypeStr=boolean
  Memory : Memory
  Multiport Switch : MultiPortSwitch  DataPortOrder=Zero-based contiguous  Inputs=7  DataPortForDefault=Additional data port  zeroidx=on
  Mux : Mux
  Relational Operator : RelationalOperator  Operator===  OutDataTypeStr=boolean
  Saturation : Saturate  LowerLimit=0
  Timer : Subsystem
  To Workspace2 : ToWorkspace  VariableName=Gear  SampleTime=t_sample  SaveFormat=Array
  Transport Delay2 : TransportDelay  DelayTime=0.3  BufferSize=10000
  ig_new : Subsystem  TreatAsAtomicUnit=on
  ig_prev : Subsystem  TreatAsAtomicUnit=on
  linear_interp : Fcn  Expr=u(2)+u(1)*(u(3)-u(2))/u(4)
  Gear_ratio : Outport
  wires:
  BUS_Control/1 -> Bus Selector1/1
  Transport Delay2/1 -> Detect Change1/1, Memory/1, ig_new/1(ig), Detect Change/1
  Saturation/1 -> Mux/1
  Logical Operator/1 -> Timer/1(Set)
  Detect Change1/1 -> Timer/2(Reset)
  Relational Operator/1 -> Logical Operator/1
  linear_interp/1 -> Gear_ratio/1, Relational Operator/2  "Gear_ratio [-]"
  Constant7/1 -> Mux/4
  Data Store Read/1 -> Mux/3
  Data Store Read1/1 -> Mux/2, Relational Operator/1
  Timer/1(Count) -> Saturation/1
  Memory/1 -> ig_prev/1(ig)
  Detect Change/1 -> ig_prev/Trigger, ig_new/Trigger
  Mux/1 -> linear_interp/1
  Constant/1 -> Multiport Switch/9, Multiport Switch/2
  Constant6/1 -> Multiport Switch/8
  Constant5/1 -> Multiport Switch/7
  Constant4/1 -> Multiport Switch/6
  Constant3/1 -> Multiport Switch/5
  Constant2/1 -> Multiport Switch/4
  Constant1/1 -> Multiport Switch/3
  Bus Selector1/1 -> Multiport Switch/1, To Workspace2/1  "<Gear[-]>"
  Multiport Switch/1 -> Transport Delay2/1

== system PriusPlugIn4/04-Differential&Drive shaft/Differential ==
  Tgd : Inport
  T_drv_sft : Inport  Port=2
  Gain : Gain  Gain=Differential.ig(1)
  Sum5 : Sum  Inputs=+-|
  inertia rear drive shaft : Gain  Gain=1/Differential.Inertia
  ratio target gear : Gain  Gain=Differential.ig(1)
  "to_angle " : Integrator  InitialCondition=om_diff_ic
  om_diff : Outport
  om_diff*ig : Outport  Port=2
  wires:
  Gain/1 -> om_diff*ig/1
  Tgd/1 -> ratio target gear/1
  ratio target gear/1 -> Sum5/1  "T_outp_sft_i"
  "to_angle "/1 -> Gain/1, om_diff/1  "om_diff [rad/s]"
  Sum5/1 -> inertia rear drive shaft/1
  inertia rear drive shaft/1 -> "to_angle "/1  "omp_diff"
  T_drv_sft/1 -> Sum5/2  "T_drv_sft"

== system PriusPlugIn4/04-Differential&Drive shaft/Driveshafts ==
  om_diff : Inport
  BUS_Vehicle : Inport  Port=2
  Add4 : Sum  Inputs=+-
  Add5 : Sum
  Bus Selector1 : BusSelector  OutputSignals=om_wheel_f
  Integrator3 : Integrator
  To Workspace1 : ToWorkspace  VariableName=T_drvsft  SampleTime=t_sample  SaveFormat=Array
  b_cg : Gain  Gain=Driveshaft.Left.b+Driveshaft.Right.b
  k_cg : Gain  Gain=Driveshaft.Left.c+Driveshaft.Right.c
  T_drvsft : Outport
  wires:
  BUS_Vehicle/1 -> Bus Selector1/1
  om_diff/1 -> Add4/1
  Add5/1 -> T_drvsft/1, To Workspace1/1  "T_drvsft"
  b_cg/1 -> Add5/2
  k_cg/1 -> Add5/1
  Integrator3/1 -> k_cg/1
  Add4/1 -> Integrator3/1, b_cg/1
  Bus Selector1/1 -> Add4/2  "<om_wheel_f>"

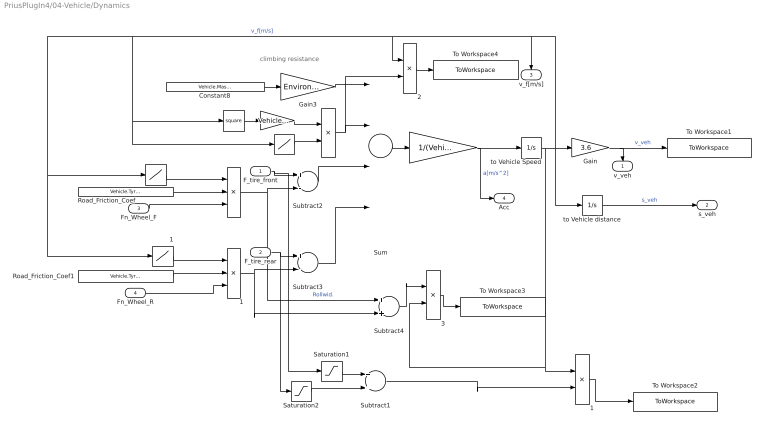
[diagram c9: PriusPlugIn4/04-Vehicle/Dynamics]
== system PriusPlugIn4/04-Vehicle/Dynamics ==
  note: climbing resistance
  F_tire_front : Inport
  F_tire_rear : Inport  Port=2
  Fn_Wheel_F : Inport  Port=3
  Fn_Wheel_R : Inport  Port=4
  "  " : Gain  Gain=1/(Vehicle.Mass+Vehicle.Load)
  "     " : Gain  Gain=Vehicle.cx*Vehicle.AreaF*Environment.Air.ro*0.5
  "      " : Math  Operator=square
  "        " : Product  Inputs=***
  "         " : Lookup  InputValues=[-1 -0.01 0 0.01 1]  Table=[-1 -1 0 1 1]
            {,1..3} (4 alike) : Product  Inputs=**
  "            " : Lookup  InputValues=[-1 -0.01 0 0.01 1]  Table=[-1 -1 0 1 1]
  "         1" : Lookup  InputValues=[-1 -0.01 0 0.01 1]  Table=[-1 -1 0 1 1]
  "        1" : Product  Inputs=***
  Constant8 : Constant  Value=Vehicle.Mass+Vehicle.Load
  Gain : Gain  Gain=3.6
  Gain3 : Gain  Gain=Environment.g*sin(Environment.Road.Incline)
  Road_Friction_Coef : Constant  Value=Vehicle.Tyre.Front.f
  Road_Friction_Coef1 : Constant  Value=Vehicle.Tyre.Rear.f
  Saturation1 : Saturate  UpperLimit=inf  LowerLimit=0
  Saturation2 : Saturate  UpperLimit=inf  LowerLimit=0
  Subtract1 : Sum
  Subtract2 : Sum  Inputs=+-
  Subtract3 : Sum  Inputs=+-
  Subtract4 : Sum
  Sum : Sum  Inputs=|-|-|+|+
  To Workspace1 : ToWorkspace  VariableName=v_vehicle  SampleTime=t_sample  SaveFormat=Array
  To Workspace2 : ToWorkspace  VariableName=P_vehicle  SampleTime=t_sample  SaveFormat=Array
  To Workspace3 : ToWorkspace  VariableName=P_roll  SampleTime=t_sample  SaveFormat=Array
  To Workspace4 : ToWorkspace  VariableName=P_air  SampleTime=t_sample  SaveFormat=Array
  to Vehicle Speed : Integrator  InitialCondition=vf0
  to Vehicle distance : Integrator  InitialCondition=vf0
  v_veh : Outport
  s_veh : Outport  Port=2
  v_f[m/s] : Outport  Port=3
  Acc : Outport  Port=4
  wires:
  "          3"/1 -> To Workspace3/1
  Subtract4/1 -> "          3"/1
  "          2"/1 -> To Workspace4/1
  Subtract1/1 -> "          1"/2
  "          1"/1 -> To Workspace2/1
  Sum/1 -> "  "/1
  "      "/1 -> "     "/1
  "         "/1 -> "        "/1
  Road_Friction_Coef/1 -> "        "/2
  "          "/1 -> "          2"/2, Sum/2
  "     "/1 -> "          "/1
  "            "/1 -> "          "/2
  "  "/1 -> to Vehicle Speed/1, Acc/1  "a[m/s^2]"
  to Vehicle Speed/1 -> "          3"/2, "          1"/1, Gain/1, to Vehicle distance/1, "          2"/1, "      "/1, "            "/1, "         "/1, "         1"/1, v_f[m/s]/1  "v_f[m/s]"
  Gain/1 -> To Workspace1/1, v_veh/1  "v_veh"
  Subtract2/1 -> Sum/3
  "        "/1 -> Subtract4/1, Subtract2/2  "Rollwid."
  "         1"/1 -> "        1"/1
  Road_Friction_Coef1/1 -> "        1"/2
  Subtract3/1 -> Sum/4
  "        1"/1 -> Subtract4/2, Subtract3/2
  Constant8/1 -> Gain3/1
  Gain3/1 -> Sum/1
  to Vehicle distance/1 -> s_veh/1  "s_veh"
  F_tire_front/1 -> Saturation1/1, Subtract2/1
  Fn_Wheel_F/1 -> "        "/3
  F_tire_rear/1 -> Saturation2/1, Subtract3/1
  Fn_Wheel_R/1 -> "        1"/3
  Saturation1/1 -> Subtract1/1
  Saturation2/1 -> Subtract1/2

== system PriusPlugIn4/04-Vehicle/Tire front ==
  v_f : Inport
  T_drsft : Inport  Port=2
  "            " : Gain  Gain=2
  "            1" : Gain  Gain=Vehicle.Tyre.Front.c
  "            2" : Gain  Gain=Vehicle.Tyre.Front.Rdyn
  "            3" : Gain  Gain=Vehicle.Tyre.Front.b
  Sum1 : Sum  Inputs=2
  Sum10 : Sum  Inputs=+-
  To Workspace1 : ToWorkspace  VariableName=om_wheel  SampleTime=t_sample  SaveFormat=Array
  Wheel : Subsystem
  "to Rot Speed     " : Integrator
  F_tire : Outport
  om_wheel : Outport  Port=2
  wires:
  T_drsft/1 -> Wheel/2(T_drsft)  "T_drv_sft"
  "            "/1 -> F_tire/1  "F_tire [N]"
  Sum1/1 -> "            "/1, Wheel/1(F_tire)  "[N]"
  Wheel/1(om_wheel) -> "            2"/1, om_wheel/1, To Workspace1/1  "om_wheel [1/s]"
  v_f/1 -> Sum10/2
  "to Rot Speed     "/1 -> "            1"/1
  "            2"/1 -> Sum10/1
  Sum10/1 -> "to Rot Speed     "/1, "            3"/1
  "            1"/1 -> Sum1/1  "[N]"
  "            3"/1 -> Sum1/2

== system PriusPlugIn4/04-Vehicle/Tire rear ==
  v_f : Inport
  T_drsft : Inport  Port=2
  "            " : Gain  Gain=2
  "            1" : Gain  Gain=Vehicle.Tyre.Front.c
  "            2" : Gain  Gain=Vehicle.Tyre.Front.Rdyn
  "            3" : Gain  Gain=Vehicle.Tyre.Front.b
  Sum1 : Sum  Inputs=2
  Sum10 : Sum  Inputs=+-
  To Workspace1 : ToWorkspace  VariableName=om_wheel2  SampleTime=t_sample  SaveFormat=Array
  Wheel : Subsystem
  "to Rot Speed     " : Integrator
  F_tire : Outport
  om_wheel : Outport  Port=2
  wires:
  "            3"/1 -> Sum1/2
  "            1"/1 -> Sum1/1  "[N]"
  Sum10/1 -> "            3"/1, "to Rot Speed     "/1
  "            2"/1 -> Sum10/1
  "to Rot Speed     "/1 -> "            1"/1
  v_f/1 -> Sum10/2
  Wheel/1(om_wheel) -> "            2"/1, To Workspace1/1, om_wheel/1  "om_wheel [1/s]"
  Sum1/1 -> Wheel/1(F_tire), "            "/1  "[N]"
  "            "/1 -> F_tire/1  "F_tire [N]"
  T_drsft/1 -> Wheel/2(T_drsft)  "T_drv_sft"

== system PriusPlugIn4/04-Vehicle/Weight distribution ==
  acc : Inport
  Constant : Constant  Value=Vehicle.Mass+Vehicle.Load
  Constant1 : Constant  Value=Vehicle.COG.Front
  Constant2 : Constant  Value=Vehicle.COG.Rear
  Constant3 : Constant  Value=Environment.g
  Constant4 : Constant  Value=Vehicle.COG.Height
  Divide : Product  Inputs=*/
  G*vzdalenost od predni napr. : Product
  Gain1 : Gain  Gain=cos(Environment.Road.Incline)
  Gain2 : Gain  Gain=sin(Environment.Road.Incline)
  Memory : Memory  X0=Vehicle.Mass/2
  Memory1 : Memory  X0=Vehicle.Mass/2
  Subtract : Sum  Inputs=+++
  Subtract1 : Sum  Inputs=+-
  Sum1 : Sum
  To Workspace2 : ToWorkspace  VariableName=Fn_Wheel_R  SampleTime=t_sample  SaveFormat=Array
  To Workspace3 : ToWorkspace  VariableName=Fn_Wheel_F  SampleTime=t_sample  SaveFormat=Array
  m*a*vyska teziste : Product  Inputs=3
  m*g : Product
  m*g1 : Product
  Fn_Wheel_F : Outport
  Fn_Wheel_R : Outport  Port=2
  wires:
  Subtract1/1 -> Memory/1
  Divide/1 -> Subtract1/2, Memory1/1
  Subtract/1 -> Divide/1
  m*g/1 -> G*vzdalenost od predni napr./1, Subtract1/1, m*g1/2
  G*vzdalenost od predni napr./1 -> Gain1/1
  m*a*vyska teziste/1 -> Subtract/1
  Constant4/1 -> m*a*vyska teziste/3, m*g1/1
  Sum1/1 -> Divide/2
  Constant2/1 -> Sum1/2
  Constant1/1 -> Sum1/1, G*vzdalenost od predni napr./2
  Constant3/1 -> m*g/2
  Constant/1 -> m*g/1, m*a*vyska teziste/2
  Memory/1 -> To Workspace3/1, Fn_Wheel_F/1
  Memory1/1 -> To Workspace2/1, Fn_Wheel_R/1
  Gain1/1 -> Subtract/2
  m*g1/1 -> Gain2/1
  Gain2/1 -> Subtract/3
  acc/1 -> m*a*vyska teziste/1

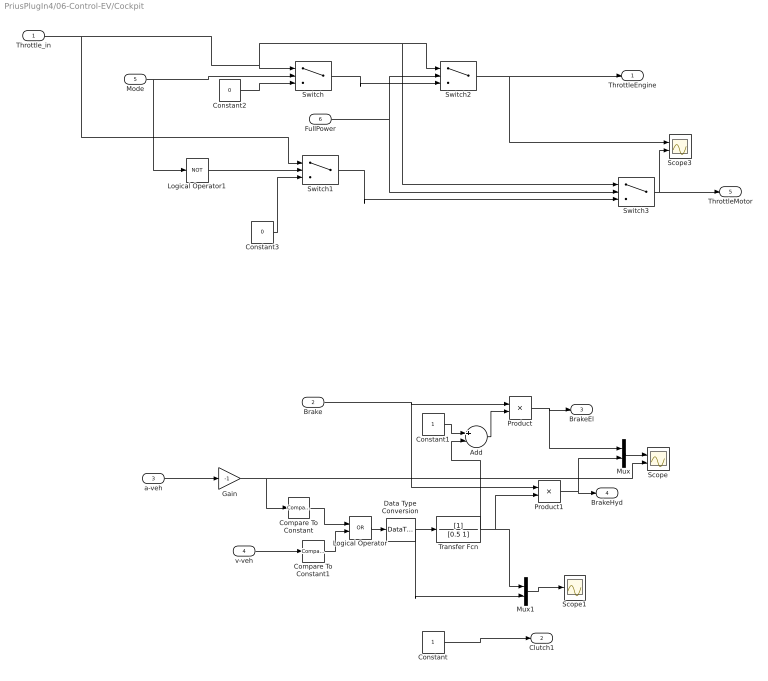
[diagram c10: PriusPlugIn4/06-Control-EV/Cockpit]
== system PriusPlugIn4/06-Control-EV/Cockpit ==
  Throttle_in : Inport
  Brake : Inport  Port=2
  a-veh : Inport  Port=3
  v-veh : Inport  Port=4
  Mode : Inport  Port=5
  FullPower : Inport  Port=6
  Add : Sum  Inputs=+-
  Compare To Constant : simulink/Logic and Bit Operations/Compare To Constant  relop=>=  const=1.5  OutDataTypeStr=uint8
  Compare To Constant1 : simulink/Logic and Bit Operations/Compare To Constant  relop=<=  const=3  OutDataTypeStr=uint8
  Constant : Constant
  Constant1 : Constant
  Constant2 : Constant  Value=0
  Constant3 : Constant  Value=0
  Data Type Conversion : DataTypeConversion
  Gain : Gain  Gain=-1
  Logical Operator : Logic  Operator=OR  AllPortsSameDT=off  OutDataTypeStr=boolean
  Logical Operator1 : Logic  Operator=NOT  AllPortsSameDT=off  OutDataTypeStr=boolean
  Mux : Mux  Inputs=2
  Mux1 : Mux  Inputs=2
  Product : Product
  Product1 : Product
  Scope : Scope  NumInputPorts=2
  Scope1 : Scope
  Scope3 : Scope  NumInputPorts=2
  Switch{,1..3} (4 alike) : Switch  Threshold=1
  Transfer Fcn : TransferFcn  Denominator=[0.5 1]
  ThrottleEngine : Outport
  Clutch1 : Outport  Port=2
  BrakeEl : Outport  Port=3
  BrakeHyd : Outport  Port=4
  ThrottleMotor : Outport  Port=5
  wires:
  Constant/1 -> Clutch1/1
  Product/1 -> BrakeEl/1, Mux/1
  Brake/1 -> Product/1, Product1/1
  Product1/1 -> BrakeHyd/1, Mux/2
  Mux/1 -> Scope/1
  a-veh/1 -> Gain/1
  Add/1 -> Product/2
  Constant1/1 -> Add/1
  Gain/1 -> Scope/2, Compare To Constant/1
  Compare To Constant/1 -> Logical Operator/1
  v-veh/1 -> Compare To Constant1/1
  Compare To Constant1/1 -> Logical Operator/2
  Logical Operator/1 -> Data Type Conversion/1
  Transfer Fcn/1 -> Mux1/1, Product1/2, Add/2
  Data Type Conversion/1 -> Transfer Fcn/1, Mux1/2
  Mux1/1 -> Scope1/1
  Constant2/1 -> Switch/3
  Mode/1 -> Switch/2, Logical Operator1/1
  Logical Operator1/1 -> Switch1/2
  Constant3/1 -> Switch1/3
  Switch/1 -> Switch2/3
  Switch1/1 -> Switch3/3
  FullPower/1 -> Switch2/2, Switch3/2
  Switch2/1 -> ThrottleEngine/1, Scope3/1
  Switch3/1 -> Scope3/2, ThrottleMotor/1
  Throttle_in/1 -> Switch1/1, Switch/1, Switch3/1, Switch2/1

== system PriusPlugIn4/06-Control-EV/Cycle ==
  Acc : Step  Time=15  After=250  SampleTime=0
  Constant1 : Constant
  Constant2 : Constant  Value=2
  Demux : Demux  Outputs=2
  From File : FromFile  FileName=NEDC.mat  ExtrapolationBeforeFirstDataPoint=Hold first value  ExtrapolationAfterLastDataPoint=Hold last value  SampleTime=0.1
  From File1 : FromFile  FileName=artemis_mw130.mat  ExtrapolationBeforeFirstDataPoint=Hold first value  ExtrapolationAfterLastDataPoint=Hold last value  SampleTime=0.1
  From File2 : FromFile  FileName=artemis_URM150.mat  ExtrapolationBeforeFirstDataPoint=Hold first value  ExtrapolationAfterLastDataPoint=Hold last value  SampleTime=0.1
  Multiport Switch : MultiPortSwitch  Inputs=4  zeroidx=off
  Terminator : Terminator
  To Workspace : ToWorkspace  VariableName=v_dem  SampleTime=t_sample  SaveFormat=Array
  To Workspace2 : ToWorkspace  VariableName=Gear_dem  SampleTime=t_sample  SaveFormat=Array
  Gear_dem [-] : Outport
  v_dem [-] : Outport  Port=2
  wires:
  Constant1/1 -> Gear_dem [-]/1, To Workspace2/1
  From File/1 -> Demux/1
  Constant2/1 -> Multiport Switch/1
  Multiport Switch/1 -> To Workspace/1, v_dem [-]/1
  Demux/1 -> Multiport Switch/2
  From File2/1 -> Multiport Switch/3
  From File1/1 -> Multiport Switch/4
  Acc/1 -> Multiport Switch/5
  Demux/2 -> Terminator/1
